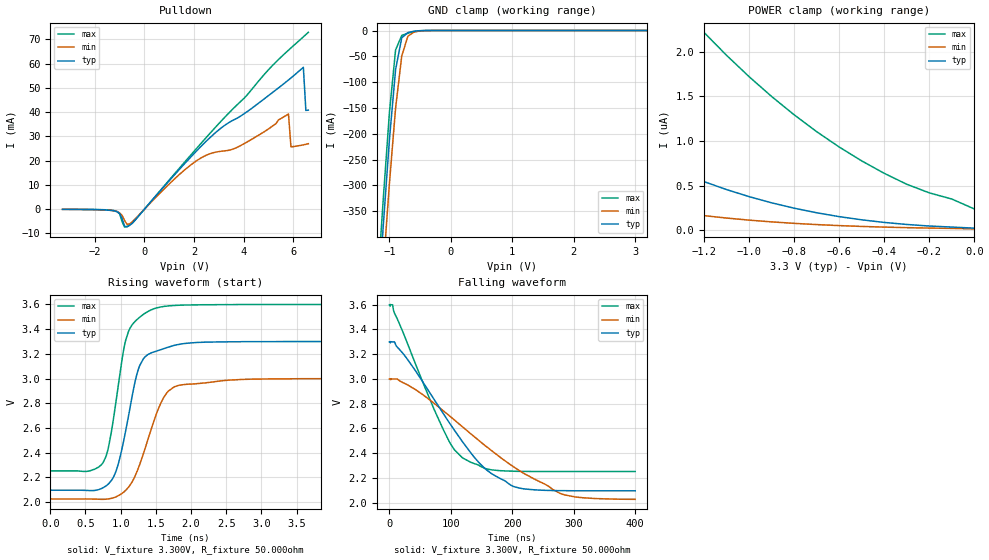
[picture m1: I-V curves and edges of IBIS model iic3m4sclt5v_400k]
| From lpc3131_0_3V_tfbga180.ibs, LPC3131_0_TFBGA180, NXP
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| iic3m4sclt5v
|   IIC Pad
|   Serial Clock Signal
| Normal 400 kHz Open-drain Mode (ehs=0, encs=0)
[Model]   iic3m4sclt5v_400k | of iic3m4sclt5v
Model_type   I/O_open_drain
Polarity   Non-Inverting
|  Reciever Thresholds
Vinl   = 0.99V
Vinh   = 2.31V
| AC Test Load Conditions
Vref   = 0
Cref   = 0
Rref   = 1000000000
Vmeas   = 1.65
| [Process Range]   typical   min   max
| C_comp edge width   400.000ps   400.000ps   400.000ps
| C_comp Tstrobe   40.000fs   40.000fs   40.000fs
C_comp   1.627pF   1.571pF   1.694pF
[Temperature Range]   25   125   -40
[Voltage Range]   3.30V   3.00V   3.60V
[GND Clamp Reference]   0.00V   0.00V   0.00V
[Pulldown Reference]   0.00V   0.00V   0.00V
[POWER Clamp Reference]   3.30V   3.00V   3.60V
[Pullup Reference]   3.30V   3.00V   3.60V
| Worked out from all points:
|   slope of the pulldown table from 0 to 0.495 V, typ, clamps not added: 84.6 ohm
|   GND clamp passes 1 mA (typ) near -0.57 V on its own axis
|   rising waveform, V_fixture 3.300V, R_fixture 50.000ohm: 20-80 % time 263ps typ, 362ps min, 230ps max; typ from 2.1 V to 3.3 V
|   falling waveform, V_fixture 3.300V, R_fixture 50.000ohm: 20-80 % time 100ns typ, 152ns min, 68.7ns max; typ from 3.3 V to 2.1 V
[GND Clamp]
| ref voltage   0.00V   0.00V   0.00V
|   Voltage   I(typ)   I(min)   I(max)
-3.3V     -4.643A    -4.695A    -4.614A
-1.2V     -555.7mA   -637.3mA   -505.9mA
-1.1V     -377.4mA   -461.5mA   -325.3mA
-1V       -211.1mA   -295.8mA   -158.4mA
-900mV    -75.75mA   -150.4mA   -37.68mA
-800mV    -14.14mA   -49.49mA   -9.569mA
-700mV    -4.026mA   -11.01mA   -5.191mA
-600mV    -1.318mA   -2.976mA   -2.281mA
-500mV    -260.9uA   -616.2uA   -536.9uA
3.2V      14.3nA     24.62nA    32.14nA
[Power Clamp]   | Vtable = Vcc - Vpad
| ref voltage   3.30V   3.00V   3.60V
|   Voltage   I(typ)   I(min)   I(max)
-3.3V     5.245uA    2.002uA    29.68uA
-3.1V     4.436uA    1.702uA    22.91uA
-2.8V     3.477uA    1.307uA    15.06uA
-2.3V     2.236uA    785.6nA    7.494uA
-2V       1.641uA    549.3nA    5.219uA
-1.7V     1.148uA    366nA      3.8uA
-1.5V     874.4nA    270.7nA    3.094uA
-1.2V     544.7nA    163.9nA    2.215uA
-900mV    307.4nA    93.98nA    1.498uA
-600mV    152.7nA    52.35nA    932.3nA
-300mV    65.03nA    29.37nA    514.9nA
0V        23.89nA    15.31nA    238.6nA
[Pulldown]
| ref voltage   0.00V   0.00V   0.00V
|   Voltage   I(typ)   I(min)   I(max)
-3.3V     -95.96uA   -104.1uA   -74.67uA
-1.2V     -777.2uA   -758uA     -659.6uA
-1V       -1.884mA   -1.532mA   -1.944mA
-800mV    -7.105mA   -4.771mA   -7.441mA
-500mV    -5.866mA   -5.302mA   -5.87mA
2.1V      24.01mA    19.96mA    25.04mA
3.8V      37.91mA    25.82mA    43.69mA
5.8V      53.26mA    39.21mA    65.53mA
5.9V      54.1mA     25.66mA    66.46mA
6.4V      58.48mA    26.5mA     71.05mA
6.5V      40.69mA    26.73mA    71.98mA
6.6V      40.8mA     26.97mA    72.91mA
[Ramp]
R_load   = 50.000ohm
|   dV/dt(typ)   dV/dt(min)   dV/dt(max)
dV/dt_r   435.098mV/250.000ps   331.224mV/360.000ps   494.921mV/200.000ps
dV/dt_f   39.651mV/11.170ns   12.007mV/7.140ns   97.185mV/13.570ns
[Rising Waveform]  | cubic spline decimation from 2501 points
V_fixture   = 3.300V
V_fixture_min = 3.000V
V_fixture_max = 3.600V
R_fixture   = 50.000ohm
|   Time   V(typ)   V(min)   V(max)
0s        2.096V     2.025V     2.252V
750ps     2.116V     2.022V     2.319V
830ps     2.149V     2.026V     2.453V
940ps     2.26V      2.044V     2.84V
1.11ns    2.693V     2.119V     3.38V
1.22ns    3.013V     2.231V     3.472V
1.32ns    3.158V     2.387V     3.519V
1.68ns    3.255V     2.9V       3.589V
3.05ns    3.299V     2.997V     3.6V
25ns      3.3V       3V         3.6V
[Falling Waveform]  | cubic spline decimation from 40001 points
V_fixture   = 3.300V
V_fixture_min = 3.000V
V_fixture_max = 3.600V
R_fixture   = 50.000ohm
|   Time   V(typ)   V(min)   V(max)
0s        3.3V       3V         3.6V
5.16ns    3.3V       3V         3.599V
42.72ns   3.064V     2.913V     3.117V
88.61ns   2.713V     2.739V     2.581V
105.8ns   2.585V     2.668V     2.427V
119ns     2.492V     2.613V     2.362V
155.3ns   2.277V     2.463V     2.277V
202.5ns   2.13V      2.288V     2.254V
285.1ns   2.097V     2.063V     2.252V
400ns     2.096V     2.027V     2.252V
